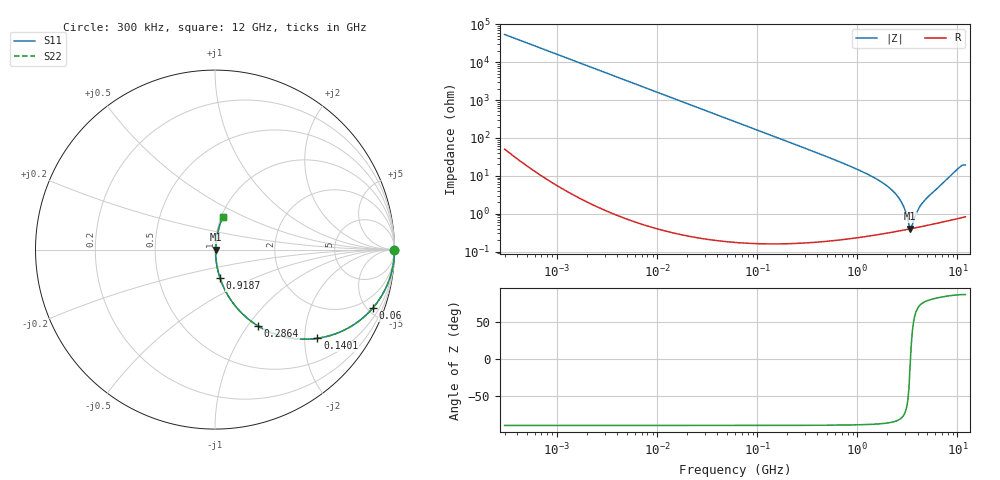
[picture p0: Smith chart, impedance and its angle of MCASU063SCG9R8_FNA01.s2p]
! MCASU063SCG9R8_FNA01  S-PARAMETER MODEL  ( General Type )
! Model Generated by TAIYO YUDEN Corporation (http://www.ty-top.com)
! Version 1.0
! TAIYO YUDEN Control No. 130801
! Copyright(c) 2013 TAIYO YUDEN CO.,LTD. All Rights Reserved.
! Product Description (link to TY-COMPAS)
! https://ds.yuden.co.jp/TYCOMPAS/or/detail?pn=MCASU063SCG9R8DFNA01&u=M
! Products Name : Multilayer Ceramic Capacitors
! Characteristics :
!  Capacitance : 9.8 pF , Rated Voltage : 50V , TCC : CG / C0G
!  Case Size : 0.6 x 0.3 / 0.024 x 0.012 [mm/inch] , Thickness : 0.3 / 0.012 [mm/inch]
!  (Conditions: Temperature = 25 degC , DC Bias Current/Voltage = 0A / 0V)
! External Node Assignments :
!  1  o---| |---o  2
! GND o---------o GND
! Frequency Range : 0.3MHz  -  12000MHz  [ 401 STEP ]
# MHz S RI R 50
! Freq[MHz].  S11 Real  S11 Imag  S21 Real  S21 Imag  S12 Real  S12 Imag  S22 Real  S22 Imag
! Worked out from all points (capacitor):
!   401 points, 300 kHz to 12 GHz, reference 50 ohm
!   read as one part in series: C = 9.84 pF near 316.3 kHz
!   lowest |Z| = 401 mohm at 3.365 GHz (marker M1)
!   series resonance near 3.392 GHz, so ESL is about 220 pH
!   S11 on the Smith chart (normalised r, x): 300 kHz: open; 60 MHz: 1.00, -5.39; 140.1 MHz: 1.00, -2.31; 286.4 MHz: 1.00, -1.12; 918.7 MHz: 1.00, -0.33; 12 GHz: 1.02, +0.38
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0.3  1 -0.00186  5.18e-06 0.00186  5.18e-06 0.00186  1 -0.00186
1.769972  0.9999 -0.0109  0.000123 0.0109  0.000123 0.0109  0.9999 -0.0109
10.44266  0.9958 -0.0643  0.00417 0.0643  0.00417 0.0643  0.9958 -0.0643
26.39317  0.974 -0.159  0.026 0.159  0.026 0.159  0.974 -0.159
60  0.8788 -0.3261  0.1212 0.3261  0.1212 0.3261  0.8788 -0.3261
89.27472  0.766 -0.4229  0.234 0.4229  0.234 0.4229  0.766 -0.4229
140.0606  0.5704 -0.4943  0.4296 0.4943  0.4296 0.4943  0.5704 -0.4943
286.3882  0.2398 -0.4255  0.7602 0.4255  0.7602 0.4255  0.2398 -0.4255
353.9943  0.1705 -0.3742  0.8295 0.3742  0.8295 0.3742  0.1705 -0.3742
918.7169  0.028 -0.1582  0.972 0.1582  0.972 0.1582  0.028 -0.1582
1480.043  0.0104 -0.0873  0.9896 0.0873  0.9896 0.0873  0.0104 -0.0873
2088.533  0.00541 -0.0476  0.9946 0.0476  0.9946 0.0476  0.00541 -0.0476
2448.343  0.00436 -0.0314  0.9956 0.0314  0.9956 0.0314  0.00436 -0.0314
2722.03  0.00399 -0.021  0.996 0.021  0.996 0.021  0.00399 -0.021
2947.191  0.00387 -0.0133  0.9961 0.0133  0.9961 0.0133  0.00387 -0.0133
3276.641  0.0039 -0.00326  0.9961 0.00326  0.9961 0.00326  0.0039 -0.00326
3364.605  0.00395 -0.000597  0.9961 0.000597  0.9961 0.000597  0.00395 -0.000597
3547.679  0.00407 0.00323  0.9959 -0.00323  0.9959 -0.00323  0.00407 0.00323
4050.141  0.0045 0.012  0.9955 -0.012  0.9955 -0.012  0.0045 0.012
4875.354  0.00541 0.0244  0.9946 -0.0244  0.9946 -0.0244  0.00541 0.0244
10236.47  0.0313 0.152  0.9687 -0.152  0.9687 -0.152  0.0313 0.152
12000  0.0428 0.1821  0.9572 -0.1821  0.9572 -0.1821  0.0428 0.1821
